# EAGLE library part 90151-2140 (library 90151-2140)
Headers & Wire Housings C-Grid PCB Conn DR V onn DR Vt Tn-A 40Ckt Source: Datasheet
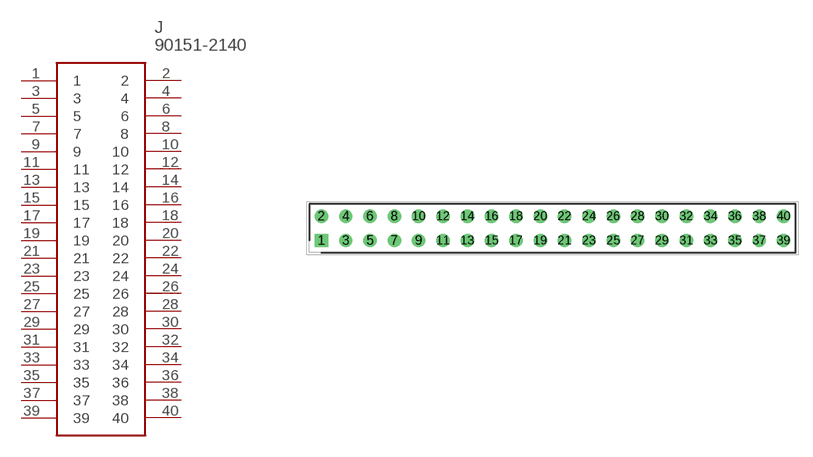
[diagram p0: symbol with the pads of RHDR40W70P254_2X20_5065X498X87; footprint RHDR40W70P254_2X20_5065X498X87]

Designator prefix J

## 90151-2140 (Description: Headers & Wire Housings C-Grid PCB Conn DR V onn DR Vt Tn-A 40Ckt; Height: 8.7mm; Manufacturer_Name: Molex; Manufacturer_Part_Number: 90151-2140; Mouser_Part_Number: 538-90151-2140; Mouser_Price-Stock: https://www.mouser.co.uk/ProductDetail/Molex/90151-2140?qs=WjPO6T6WDwtb8fg%2FDgSCUQ%3D%3D)  [RHDR40W70P254_2X20_5065X498X87]
1  1
2  2
3  3
4  4
5  5
6  6
7  7
8  8
9  9
10  10
11  11
12  12
13  13
14  14
15  15
16  16
17  17
18  18
19  19
20  20
21  21
22  22
23  23
24  24
25  25
26  26
27  27
28  28
29  29
30  30
31  31
32  32
33  33
34  34
35  35
36  36
37  37
38  38
39  39
40  40

## Footprint RHDR40W70P254_2X20_5065X498X87 (pad centres in mm)
90151-2140
drill 0.9 pad 1.35 square: 1 0,0
drill 0.9 pad 1.35: 2 0,2.54; 3 2.54,0; 4 2.54,2.54; 5 5.08,0; 6 5.08,2.54; 7 7.62,0; 8 7.62,2.54; 9 10.16,0; 10 10.16,2.54; 11 12.7,0; 12 12.7,2.54; 13 15.24,0; 14 15.24,2.54; 15 17.78,0; 16 17.78,2.54; 17 20.32,0; 18 20.32,2.54; 19 22.86,0; 20 22.86,2.54; 21 25.4,0; 22 25.4,2.54; 23 27.94,0; 24 27.94,2.54; 25 30.48,0; 26 30.48,2.54; 27 33.02,0; 28 33.02,2.54; 29 35.56,0; 30 35.56,2.54; 31 38.1,0; 32 38.1,2.54; 33 40.64,0; 34 40.64,2.54; 35 43.18,0; 36 43.18,2.54; 37 45.72,0; 38 45.72,2.54; 39 48.26,0; 40 48.26,2.54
